PROGRAM MAIN
VAR
	sMappingInHmi : STRING := '%l%Text1%/l%';
	bSwitchMapping : BOOL;
	rTrig : R_TRIG;
END_VAR

rTrig(CLK:= bSwitchMapping);

IF rTrig.Q THEN
	IF sMappingInHmi = '%l%Text1%/l%' THEN
		sMappingInHmi := '%l%Text2%/l%';
	ELSE
		sMappingInHmi := '%l%Text1%/l%';
	END_IF
END_IF

END_PROGRAM
